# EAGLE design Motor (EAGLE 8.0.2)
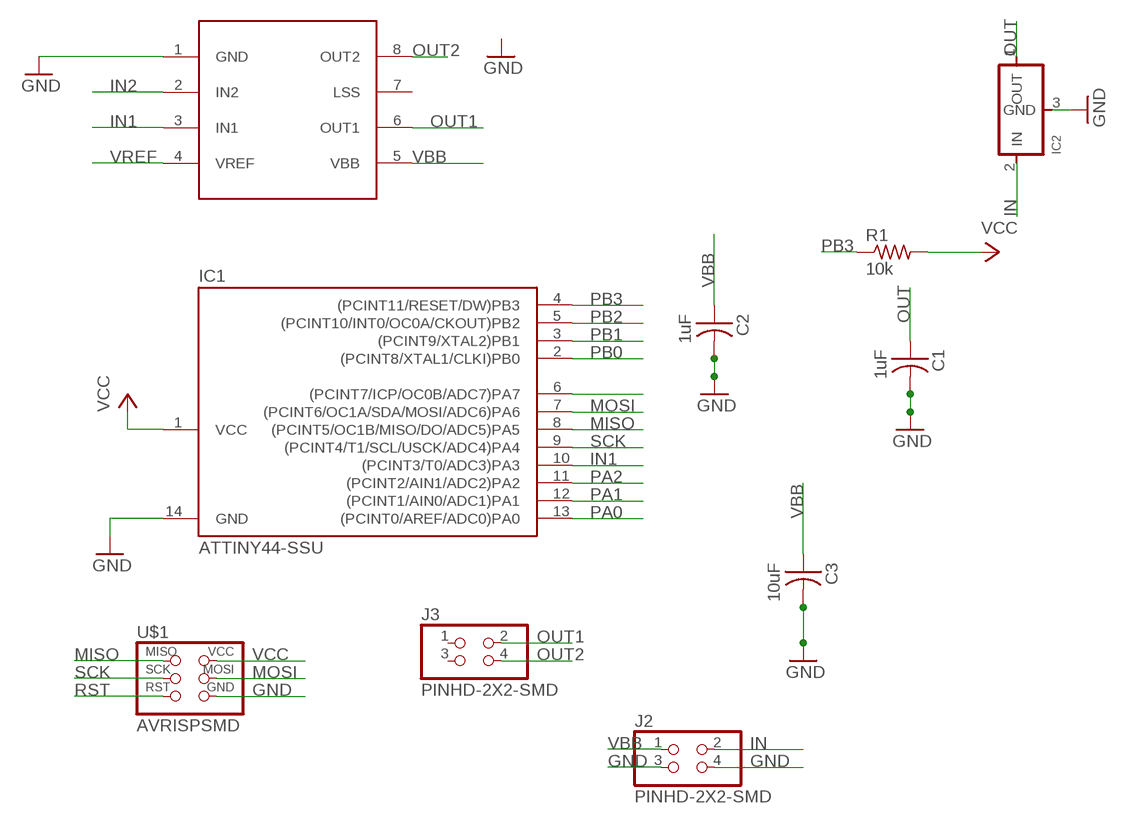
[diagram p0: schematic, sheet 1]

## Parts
C1  1uF  CAP-US1206FAB  [C1206FAB]
C2  1uF  CAP-US1206FAB  [C1206FAB]
C3  10uF  CAP-US1206FAB  [C1206FAB]
IC1  ATTINY44-SSU  [SOIC14]
IC2  REGULATORSOT23  [SOT23]
J2  PINHD-2X2-SMD  [2X02SMD]
J3  PINHD-2X2-SMD  [2X02SMD]
R1  10k  RES-US1206FAB  [R1206FAB]
U$1  AVRISPSMD  [2X03SMD]
U$3  A4953-H-BRIDGE-MOTOR-DRIVER  [SOIC8]

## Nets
GND: C1.2 C2.2 C3.2 IC1.14(GND) IC2.3(GND) J2.3 J2.4 U$1.6(GND) U$3.1(GND)
IN: IC2.2(IN) J2.2
IN1: IC1.10((PCINT3/T0/ADC3)PA3) U$3.3(IN1)
IN2: U$3.2(IN2)
MISO: IC1.8((PCINT5/OC1B/MISO/DO/ADC5)PA5) U$1.1(MISO)
MOSI: IC1.7((PCINT6/OC1A/SDA/MOSI/ADC6)PA6) U$1.4(MOSI)
N$5: IC1.6((PCINT7/ICP/OC0B/ADC7)PA7)
OUT: C1.1 IC2.1(OUT)
OUT1: J3.2 U$3.6(OUT1)
OUT2: J3.4 U$3.8(OUT2)
PA0: IC1.13((PCINT0/AREF/ADC0)PA0)
PA1: IC1.12((PCINT1/AIN0/ADC1)PA1)
PA2: IC1.11((PCINT2/AIN1/ADC2)PA2)
PB0: IC1.2((PCINT8/XTAL1/CLKI)PB0)
PB1: IC1.3((PCINT9/XTAL2)PB1)
PB2: IC1.5((PCINT10/INT0/OC0A/CKOUT)PB2)
PB3: IC1.4((PCINT11/RESET/DW)PB3) R1.1
RST: U$1.5(RST)
SCK: IC1.9((PCINT4/T1/SCL/USCK/ADC4)PA4) U$1.3(SCK)
VBB: C2.1 C3.1 J2.1 U$3.5(VBB)
VCC: IC1.1(VCC) R1.2 U$1.2(VCC)
VREF: U$3.4(VREF)
Unconnected: J3.1 J3.3 U$3.7(LSS)

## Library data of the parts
C1-C3 = fab:CAP-US
IC1 = fab:ATTINY44
IC2 = fab:REGULATOR
J2 J3 = fab:PINHD-2X2-SMD
R1 = fab:RES-US: Resistor (US Symbol)
U$1 = fab:AVRISP
U$3 = fab:A4953-H-BRIDGE-MOTOR-DRIVER

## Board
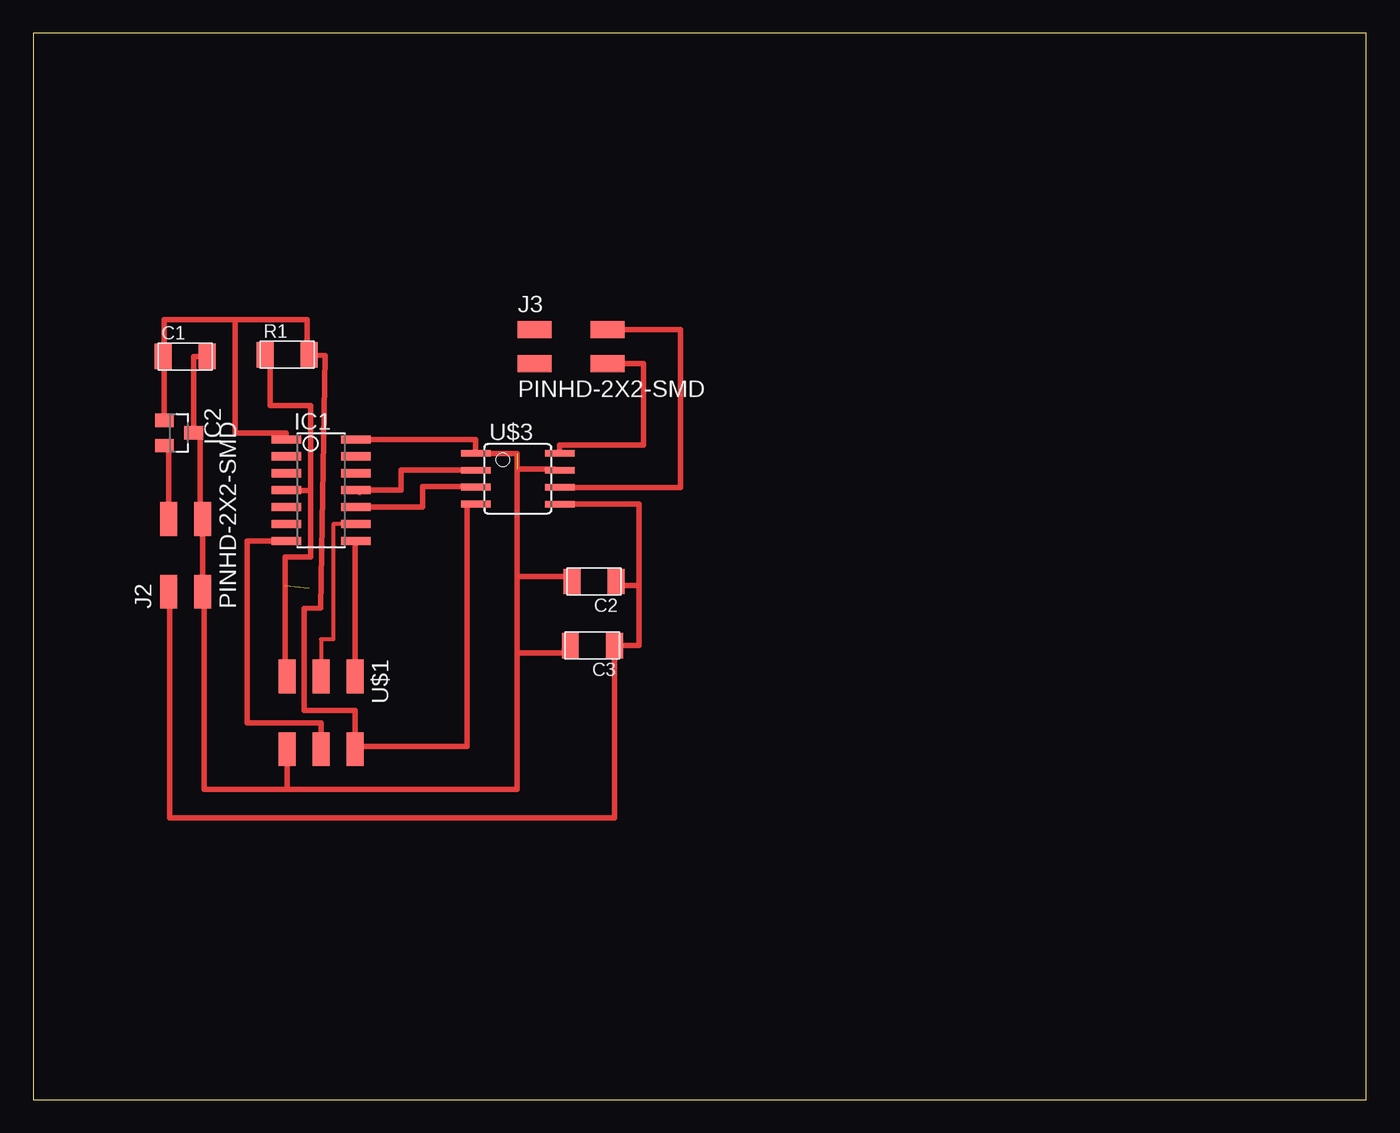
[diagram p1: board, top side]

Size 100 x 80 mm. Coordinates in mm from the lower left corner, seen from the top.
Outline: 0,0 100,0 100,80 0,80 0,0
Copper layers (1*16): Top 0.035mm / dielectric 1.5mm / Bottom 0.035mm
Design rules "default *": minimum track width 10mil, minimum drill 24mil, track to track 12mil, track to pad 12mil, pad to pad 12mil, via to via 12mil, smd to smd 12mil, copper to edge 40mil, drill to drill 8mil, minimum pad ring 10mil, minimum via ring 8mil, stop-mask expansion 4mil, vias tented up to drill 0mil, thermal gap 10mil

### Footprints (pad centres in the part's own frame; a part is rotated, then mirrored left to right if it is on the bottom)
C1206FAB = smd 1.27 x 1.905: 1 -1.651,0; 2 1.651,0
SOIC14 = smd 0.61 x 2.21: 1 -3.81,-2.603; 2 -2.54,-2.603; 3 -1.27,-2.603; 4 0,-2.603; 5 1.27,-2.603; 6 2.54,-2.603; 7 3.81,-2.603; 8 3.81,2.603; 9 2.54,2.603; 10 1.27,2.603; 11 0,2.603; 12 -1.27,2.603; 13 -2.54,2.603; 14 -3.81,2.603
SOT23 = smd 1 x 1.4: 1 -0.95,-1.1; 2 0.95,-1.1; 3 0,1.1
2X02SMD = smd 2.54 x 1.27: 1 -2.54,1.27; 2 2.92,1.27; 3 -2.54,-1.27; 4 2.92,-1.27
R1206FAB = smd 1.27 x 1.905: 1 -1.651,0; 2 1.651,0
2X03SMD = smd 2.54 x 1.27: 1 -2.54,2.54; 2 2.92,2.54; 3 -2.54,0; 4 2.92,0; 5 -2.54,-2.54; 6 2.92,-2.54
SOIC8 = smd 0.5 x 2.2: 1 -1.905,-3.154; 2 -0.645,-3.154; 3 0.625,-3.154; 4 1.895,-3.154; 5 1.905,3.154; 6 0.635,3.154; 7 -0.635,3.154; 8 -1.905,3.154

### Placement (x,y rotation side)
C1  11.38,55.75 0 top
C2  42.08,38.87 180 top
C3  41.94,34.05 180 top
IC1  21.59,45.72 270 top
IC2  10.93,50.02 270 top
J2  11.43,40.64 90 top
J3  40.16,56.49 0 top
R1  19.05,55.88 0 top
U$1  21.59,29.21 270 top
U$3  36.34,46.58 270 top

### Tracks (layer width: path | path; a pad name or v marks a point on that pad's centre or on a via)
GND  (1 unrouted)
  Top 0.406: C1.2 12.03,55.75 IC2.3 12.52,50.02 12.52,44.07 12.7,44.07 J2.4 J2.3 12.84,38.1 12.84,23.28 19.05,23.28 | 36.28,41.09 36.28,48.48 U$3.1 33.19,49.53 IC1.14 | 36.28,41.09 36.28,39.24 40.42,39.24 C2.2 | 36.28,41.09 36.29,41.09 36.29,33.52 | 36.29,33.52 40.48,33.52 40.48,33.56 40.29,33.56 C3.2 | 36.28,47.31 39.08,47.31 39.08,47.21 | 19.05,23.28 U$1.6 | 19.05,23.28 36.29,23.28 36.29,33.52
IN
  Top 0.406: IC2.2 10.16,49.07 J2.2
IN1
  Top 0.406: IC1.10 29.2,44.45 29.2,46 33.19,46 U$3.3
IN2
  Top 0.406: 24.5,45.54 24.5,45.76 24.5,45.74 27.59,45.74 27.59,47.22 U$3.2
MISO
  Top 0.406: IC1.8 24.13,41.91 U$1.1
MOSI
  Top 0.406: IC1.7 16.03,41.91 16.03,28.27 21.59,28.27 U$1.4
OUT
  Top 0.406: C1.1 9.83,55.75 IC2.1
OUT1
  Top 0.406: J3.2 48.54,57.76 48.54,45.93 U$3.6
OUT2
  Top 0.406: J3.4 45.79,55.22 45.79,49.1 39.5,49.1 U$3.8
PB3  (1 unrouted)
  Top 0.406: R1.1 17.78,55.88 17.78,52.07 20.79,52.07 20.79,45.93 | 20.79,45.93 20.79,45.71 20.75,45.71 IC1.4 | 18.89,32.32 18.89,38.58 18.89,40.71 20.79,40.71 20.79,45.93
SCK
  Top 0.305: IC1.9 22.5,43.18 22.5,34.53 21.59,34.53 U$1.3
VBB
  Top 0.406: U$3.5 45.43,44.67 45.43,38.57 | 45.43,38.57 43.73,38.57 C2.1 | 45.43,38.57 45.43,34.05 C3.1 43.59,21.15 10.24,21.15 10.24,38.1 J2.1
VCC
  Top 0.406: U$1.2 24.13,29.21 20.32,29.21 20.32,36.83 21.55,36.9 21.89,55.81 R1.2 20.55,55.88 20.55,58.53 15.16,58.53 | 15.16,58.53 15.16,50.01 18.99,50.01 IC1.1 | 15.16,58.53 9.84,58.53 9.84,55.85
VREF
  Top 0.406: U$3.4 32.55,44.68 32.55,26.48 23.88,26.48 23.88,26.39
